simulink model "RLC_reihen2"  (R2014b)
settings: Solver=ode45  StartTime=0.0  StopTime=0.005  RelTol=1e-3
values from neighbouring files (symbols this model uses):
  ampl_ug = 2    [RLC_reihen_1.m]    (also in RLC_reihen_3.m; RLC_reihen_4.m)
  Az = [-R/L, -1/L;1/C, 0]    [RLC_reihen_1.m]    (also in RLC_reihen_4.m)
  Bz = [1/L; 0]    [RLC_reihen_1.m]    (also in RLC_reihen_4.m)
  f_ug = 1000    [RLC_reihen_1.m]    (also in RLC_reihen_3.m; RLC_reihen_4.m)
  i0 = 0    [RLC_reihen_1.m]    (also in RLC_reihen_3.m; RLC_reihen_4.m)
  phi_ug = pi/3    (= 1.0471975512)    [RLC_reihen_1.m]    (also in RLC_reihen_3.m; RLC_reihen_4.m)
  uc0 = -2    [RLC_reihen_1.m]    (also in RLC_reihen_3.m; RLC_reihen_4.m)

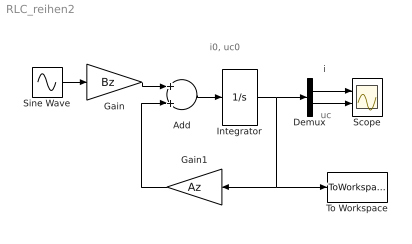
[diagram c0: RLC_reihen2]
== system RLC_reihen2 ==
  note: i0, uc0
  note: uc
  note: i
  Add : Sum
  Demux : Demux  Outputs=2
  Gain : Gain  Gain=Bz  Multiplication=Matrix(K*u)
  Gain1 : Gain  Gain=Az  Multiplication=Matrix(K*u)
  Integrator : Integrator  InitialCondition=[i0, uc0]
  Scope : Scope  NumInputPorts=2
  Sine Wave : Sin  Amplitude=ampl_ug  Frequency=2*pi*f_ug  Phase=phi_ug  SampleTime=0
  To Workspace : ToWorkspace  VariableName=x  SaveFormat=Timeseries  SampleTime=-1
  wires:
  Gain/1 -> Add/1
  Sine Wave/1 -> Gain/1
  Add/1 -> Integrator/1
  Gain1/1 -> Add/2
  Integrator/1 -> Demux/1, Gain1/1, To Workspace/1
  Demux/1 -> Scope/1
  Demux/2 -> Scope/2
